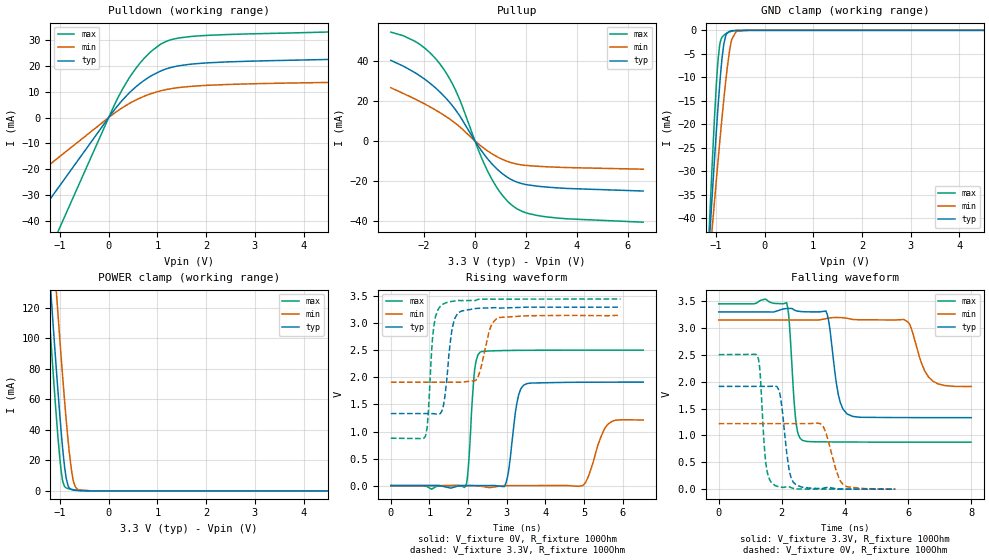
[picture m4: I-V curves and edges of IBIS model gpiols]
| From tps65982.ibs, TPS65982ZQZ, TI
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|   gpiols Model
[Model]   gpiols
Model_type   I/O
Polarity   Non-Inverting
Enable   Active-High
Vinl = 0.80
Vinh = 2.00
Vmeas = 1.65
Vref = 0
Cref = 2pF
Rref = 150
|   typ   min   max
|   (nom PVT)   (fast PVT)   (slow PVT)
C_comp   5.680e-13   5.282e-13   6.367e-13
| Where nom  PVT is Nominal Process, 3.3V, 27C
|   Fast PVT is Strong Process,  3.45V, -40C
|   Slow PVT is Weak Process,   3.15V, 125C
[Voltage Range]   3.3   3.15   3.45
|Junction Temperature
[Temperature Range]   27   125   -40
[Pullup Reference]   3.3   3.15   3.45
[Pulldown Reference]   0   0   0
[Power Clamp Reference]   3.3   3.15   3.45
[GND Clamp Reference]   0   0   0
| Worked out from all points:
|   slope of the pulldown table from 0 to 0.495 V, typ, clamps not added: 45.6 ohm
|   slope of the pullup table from 0 to 0.495 V, typ, clamps not added: 55.2 ohm
|   GND clamp passes 1 mA (typ) near -0.79 V on its own axis
|   POWER clamp passes 1 mA (typ) near -0.77 V on its own axis
|   falling waveform, V_fixture 3.3V, R_fixture 100Ohm: 20-80 % time 266ps typ, 421ps min, 167ps max; typ from 3.3 V to 1.33 V
|   rising waveform, V_fixture 0V, R_fixture 100Ohm: 20-80 % time 196ps typ, 332ps min, 127ps max; typ from 0 V to 1.91 V
|   rising waveform, V_fixture 3.3V, R_fixture 100Ohm: 20-80 % time 176ps typ, 244ps min, 138ps max; typ from 1.33 V to 3.3 V
|   falling waveform, V_fixture 0V, R_fixture 100Ohm: 20-80 % time 226ps typ, 351ps min, 161ps max; typ from 1.91 V to 0 V
[Pulldown]
|   Voltage   I(typ)   I(min)   I(max)
-3.3V     -86.79mA   -49.65mA   -140.2mA
-150.2mV  -3.949mA   -2.259mA   -6.381mA
151.8mV   3.848mA    2.174mA    6.273mA
274.2mV   6.61mA     3.748mA    10.72mA
460.5mV   10.26mA    5.846mA    16.51mA
653.4mV   13.38mA    7.655mA    21.39mA
854.7mV   15.98mA    9.168mA    25.38mA
1.178V    18.86mA    10.85mA    29.54mA
1.422V    20.03mA    11.59mA    30.81mA
2.041V    21.23mA    12.51mA    31.9mA
5.432V    22.9mA     13.9mA     33.63mA
6.6V      23.93mA    14.54mA    35.14mA
[GND Clamp]
|   Voltage   I(typ)   I(min)   I(max)
-3.3V     -444.3mA   -334.2mA   -593.3mA
-1.199V   -56.27mA   -57.44mA   -56.95mA
-1.116V   -42.03mA   -47.13mA   -37.61mA
-1.076V   -35.26mA   -42.18mA   -28.6mA
-988.5mV  -21.26mA   -31.67mA   -11.27mA
-923mV    -11.82mA   -24.06mA   -3.268mA
-838.2mV  -3.019mA   -14.83mA   -1.053mA
-720.1mV  -207.6uA   -4.451mA   -339.4uA
-671.1mV  -87.18uA   -1.876mA   -172.1uA
-581.6mV  -16.64uA   -214uA     -32.75uA
-330mV    -33.38nA   -287.3nA   -22.51nA
6.6V      0A         0A         0A
[Pullup]
|   Voltage   I(typ)   I(min)   I(max)
-3.3V     40.45mA    26.7mA     54.64mA
-2.134V   32.46mA    19.63mA    48.2mA
-1.567V   26.85mA    15.68mA    41.66mA
-1.213V   22.48mA    12.89mA    35.78mA
-626.2mV  13.14mA    7.428mA    21.6mA
146.6mV   -2.904mA   -1.612mA   -4.947mA
521.4mV   -9.378mA   -5.238mA   -15.78mA
1.053V    -16.22mA   -9.118mA   -26.93mA
1.475V    -19.73mA   -11.11mA   -32.55mA
2.005V    -21.92mA   -12.3mA    -36.12mA
2.831V    -23.2mA    -12.99mA   -38.18mA
6.6V      -25.17mA   -14.2mA    -40.81mA
[POWER Clamp]
|   Voltage   I(typ)   I(min)   I(max)
-3.3V     1.18A      1.219A     1.164A
-1.256V   161.6mA    213mA      130.4mA
-1.238V   153.1mA    204.6mA    121.8mA
-1.137V   106.8mA    158.3mA    75.38mA
-1.076V   79.81mA    130.9mA    48.94mA
-970.2mV  36.57mA    84.99mA    11.46mA
-940.2mV  26mA       72.61mA    5.769mA
-871.2mV  7.9mA      45.83mA    1.94mA
-812.5mV  2.002mA    26.11mA    1.349mA
-735.9mV  655.8uA    8.132mA    838.7uA
-625.7mV  235.2uA    675.5uA    309.9uA
6.6V      0A         0A         0A
[Ramp]
R_load = 100
|   typ   min   max
dV/dt_r   1.14825/1.93794e-10  0.732138/3.3001e-10   1.50297/1.27062e-10
dV/dt_f   1.1811/2.62991e-10   0.742822/4.15211e-10   1.54452/1.66157e-10
[Falling Waveform]
V_fixture = 3.3V
V_fixture_min = 3.15V
V_fixture_max = 3.45V
R_fixture = 100Ohm
|   Time   V(typ)   V(min)   V(max)
0s        3.3V       3.15V      3.45V
2.15ns    3.364V     3.15V      3.472V
2.444ns   3.324V     3.15V      1.272V
2.666ns   3.305V     3.15V      906.1mV
3.402ns   3.311V     3.176V     880.4mV
3.788ns   1.766V     3.196V     878.8mV
4.072ns   1.399V     3.181V     877.7mV
5.868ns   1.333V     3.159V     875.9mV
6.648ns   1.332V     2.09V      875.9mV
8ns       1.332V     1.912V     875.8mV
[Rising Waveform]
V_fixture = 0V
V_fixture_min = 0V
V_fixture_max = 0V
R_fixture = 100Ohm
|   Time   V(typ)   V(min)   V(max)
0s        2.643nV    40.72nV    1.626nV
1.928ns   -739.5uV   475.1uV    -18.23mV
2.004ns   -539.9uV   775.5uV    329.8mV
2.172ns   -337.2uV   -2.376mV   2.165V
2.312ns   -255.9uV   -11.24mV   2.47V
2.946ns   -10.16mV   -384.1uV   2.498V
3.434ns   1.857V     -229.2uV   2.502V
4.966ns   1.911V     26.54uV    2.505V
5.62ns    1.913V     1.139V     2.505V
6.528ns   1.913V     1.214V     2.505V
[Rising Waveform]
V_fixture = 3.3V
V_fixture_min = 3.15V
V_fixture_max = 3.45V
R_fixture = 100Ohm
|   Time   V(typ)   V(min)   V(max)
0s        1.331V     1.912V     875.8mV
894ps     1.332V     1.912V     912.6mV
962ps     1.332V     1.912V     1.265V
1.114ns   1.329V     1.912V     2.956V
1.348ns   1.434V     1.912V     3.354V
1.596ns   2.938V     1.912V     3.409V
1.824ns   3.228V     1.911V     3.422V
2.256ns   3.278V     2.013V     3.443V
2.766ns   3.289V     3.094V     3.449V
5.942ns   3.3V       3.151V     3.45V
[Falling Waveform]
V_fixture = 0V
V_fixture_min = 0V
V_fixture_max = 0V
R_fixture = 100Ohm
|   Time   V(typ)   V(min)   V(max)
0s        1.914V     1.22V      2.505V
1.234ns   1.914V     1.22V      2.474V
1.508ns   1.914V     1.22V      420.6mV
1.784ns   1.921V     1.22V      68.19mV
1.966ns   1.687V     1.22V      38.31mV
2.26ns    284mV      1.22V      37.94mV
2.456ns   77.15mV    1.22V      6.124mV
3.318ns   17.35mV    1.158V     845.4uV
3.978ns   1.772mV    68.99mV    389uV
5.596ns   221.6uV    3.548mV    99.53uV
